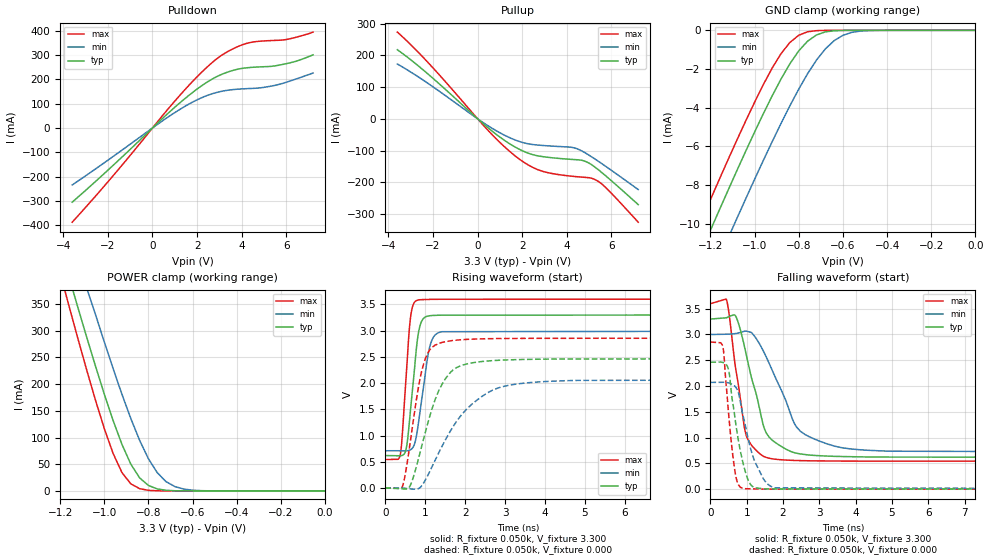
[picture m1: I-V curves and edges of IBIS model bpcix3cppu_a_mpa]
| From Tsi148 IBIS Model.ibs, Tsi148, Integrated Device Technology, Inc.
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|   MODEL bpcix3cppu_a_mpa
[Model]   bpcix3cppu_a_mpa
Model_type   I/O
Vinl  = 0.8V
Vinh  = 2.0V
Vref  = 0.0V
Rref  = 1k
Cref  = 10pF
Vmeas = 1.4V
| Values for delay from A to PAD (Tdo) are determined using
| Vref, Cref, Rref, and Vmeas.
|   INPUT TRANSITION ON DRIVER INPUT = 0.1ns
|   typ   min   max
| Tdo (rise)   1.26n   0.87n   1.86n
| Tdo (fall)   1.46n   0.99n   2.22n
|   INPUT TRANSITION ON DRIVER INPUT = 1.0ns
|   typ   min   max
| Tdo (rise)   1.28n   0.86n   1.92n
| Tdo (fall)   1.61n   1.15n   2.37n
|   typ   min   max
C_comp   2.58pF   2.53pF  2.63pF
[Temperature Range]   50.00   125.00   0.00
[Voltage Range]   3.300   3.000   3.600
|   typ   min   max
|[Supply]   VDD   1.80   1.65   1.95
|[Supply]   VDD330   3.30   3.00   3.60
[Add Submodel]
| Submodel Name   Mode
Up.bpcix3cppu_a.mpa   Non-Driving
Dn.bpcix3cppu_a.mpa   Non-Driving
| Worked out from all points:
|   slope of the pulldown table from 0 to 0.495 V, typ, clamps not added: 11.5 ohm
|   slope of the pullup table from 0 to 0.495 V, typ, clamps not added: 16.5 ohm
|   GND clamp passes 1 mA (typ) near -0.80 V on its own axis
|   POWER clamp passes 1 mA (typ) near -0.71 V on its own axis
|   rising waveform, R_fixture 0.050k, V_fixture 3.300: 20-80 % time 204ps typ, 255ps min, 159ps max; typ from 0.618 V to 3.3 V
|   falling waveform, R_fixture 0.050k, V_fixture 3.300: 20-80 % time 559ps typ, 868ps min, 364ps max; typ from 3.3 V to 0.618 V
|   rising waveform, R_fixture 0.050k, V_fixture 0.000: 20-80 % time 609ps typ, 1.09ns min, 365ps max; typ from 0 V to 2.46 V
|   falling waveform, R_fixture 0.050k, V_fixture 0.000: 20-80 % time 341ps typ, 473ps min, 227ps max; typ from 2.46 V to 0 V
[Pullup]   | Note: Vtable = Vcc - Vout
| Voltage   I(typ)   I(min)   I(max)
-3.6V     217.8mA    172.7mA    273.5mA
-2.04V    129.9mA    102.7mA    163.5mA
380mV     -23.3mA    -18.01mA   -29.87mA
1.04V     -59.81mA   -45.69mA   -77.37mA
1.7V      -89.81mA   -67.28mA   -117.9mA
2.36V     -110.6mA   -79.96mA   -149.1mA
2.91V     -119.2mA   -84.03mA   -165.5mA
4.34V     -128.6mA   -91.85mA   -181.9mA
4.89V     -136mA     -110.3mA   -185.1mA
5.33V     -156.1mA   -130.2mA   -194.1mA
5.88V     -188.2mA   -156.8mA   -226.5mA
7.2V      -270.6mA   -223.1mA   -326mA
[Pulldown]   | Note: Vtable = Vout
| Voltage   I(typ)   I(min)   I(max)
-3.6V     -305.7mA   -234.9mA   -388.2mA
-1.73V    -151mA     -115.1mA   -192.9mA
1.02V     86.89mA    64.49mA    112.8mA
2.01V     161mA      116.4mA    211.8mA
2.45V     188.9mA    133.8mA    251mA
2.89V     211.8mA    146.5mA    285.4mA
3.55V     235.6mA    157.4mA    323.4mA
4.21V     247.7mA    161.9mA    348.1mA
4.87V     251.8mA    165.7mA    357.7mA
5.75V     260mA      181.4mA    361.6mA
6.41V     274.2mA    200.9mA    373mA
7.2V      301.3mA    226.2mA    394.9mA
[POWER_Clamp]   | Note: Vtable = Vcc - Vout
| Voltage   I(typ)   I(min)   I(max)
-3.6V     3.946A     3.816A     4.188A
-1.2V     455.7mA    530.2mA    407.9mA
-1.16V    400.6mA    479.4mA    346.3mA
-1.12V    343.9mA    429.2mA    285.8mA
-1.08V    288.1mA    379.7mA    226.7mA
-1.04V    233.7mA    330.1mA    169.8mA
-1V       181.1mA    278.8mA    116.7mA
-920mV    86.97mA    180.7mA    34.22mA
-840mV    24.39mA    94.6mA     4.235mA
-720mV    1.176mA    17.25mA    44uA
-600mV    19uA       1.348mA    0A
0V        0A         0A         0A
[GND_Clamp]   | Note: Vtable = Vout
| Voltage   I(typ)   I(min)   I(max)
-3.6V     -76.49mA   -78.79mA   -75.06mA
-1.28V    -12.45mA   -14.94mA   -10.87mA
-1.24V    -11.4mA    -13.88mA   -9.809mA
-1.2V     -10.35mA   -12.84mA   -8.759mA
-1.12V    -8.273mA   -10.76mA   -6.689mA
-1.08V    -7.253mA   -9.729mA   -5.675mA
-920mV    -3.381mA   -5.752mA   -1.944mA
-840mV    -1.725mA   -3.901mA   -626uA
-760mV    -561uA     -2.244mA   -74uA
-640mV    -23uA      -536uA     -1uA
-520mV    0A         -38uA      0A
0V        0A         0A         0A
[Ramp]
| variable   typ   min   max
  dV/dt_r   1.48/0.61n   1.24/1.09n   1.71/0.37n
  dV/dt_f   1.61/0.56n   1.37/0.86n   1.83/0.36n
R_load = 0.05k
[Rising Waveform]
R_fixture = 0.050k
V_fixture = 3.300
V_fixture_min = 3.000
V_fixture_max = 3.600
|   time   V(typ)   V(min)   V(max)
0s        618mV      710mV      543mV
370ps     614mV      710mV      617mV
420ps     620mV      709mV      952mV
510ps     708mV      708mV      1.988V
640ps     1.551V     733mV      3.293V
740ps     2.338V     858mV      3.547V
830ps     2.953V     1.234V     3.583V
1.11ns    3.282V     2.679V     3.593V
1.42ns    3.293V     2.978V     3.596V
19.9ns    3.3V       3V         3.6V
[Falling Waveform]
R_fixture = 0.050k
V_fixture = 3.300
V_fixture_min = 3.000
V_fixture_max = 3.600
|   time   V(typ)   V(min)   V(max)
0s        3.3V       3V         3.6V
440ps     3.325V     3.005V     3.675V
710ps     3.335V     3.02V      2.271V
930ps     2.789V     3.062V     1.221V
1.01ns    2.53V      3.062V     995mV
1.46ns    1.23V      2.676V     638mV
1.62ns    1.006V     2.436V     600mV
2.37ns    698mV      1.207V     556mV
3.65ns    633mV      800mV      545mV
19.9ns    618mV      710mV      543mV
[Rising Waveform]
R_fixture = 0.050k
V_fixture = 0.000
V_fixture_min = 0.000
V_fixture_max = 0.000
|   time   V(typ)   V(min)   V(max)
0s        0V         0V         0V
420ps     -15mV      -1mV       13mV
610ps     26mV       -15mV      795mV
830ps     554mV      -12mV      1.917V
990ps     1.023V     134mV      2.433V
1.25ns    1.688V     531mV      2.723V
1.52ns    2.097V     937mV      2.79V
2.56ns    2.42V      1.813V     2.845V
3.74ns    2.453V     2.016V     2.852V
19.9ns    2.462V     2.071V     2.853V
[Falling Waveform]
R_fixture = 0.050k
V_fixture = 0.000
V_fixture_min = 0.000
V_fixture_max = 0.000
|   time   V(typ)   V(min)   V(max)
0s        2.462V     2.071V     2.853V
340ps     2.458V     2.073V     2.766V
500ps     2.312V     2.061V     1.469V
660ps     1.462V     2.005V     418mV
760ps     987mV      1.892V     102mV
900ps     502mV      1.418V     15mV
1.05ns    158mV      944mV      7mV
1.22ns    29mV       537mV      4mV
1.78ns    4mV        25mV       1mV
19.9ns    0V         0V         0V
